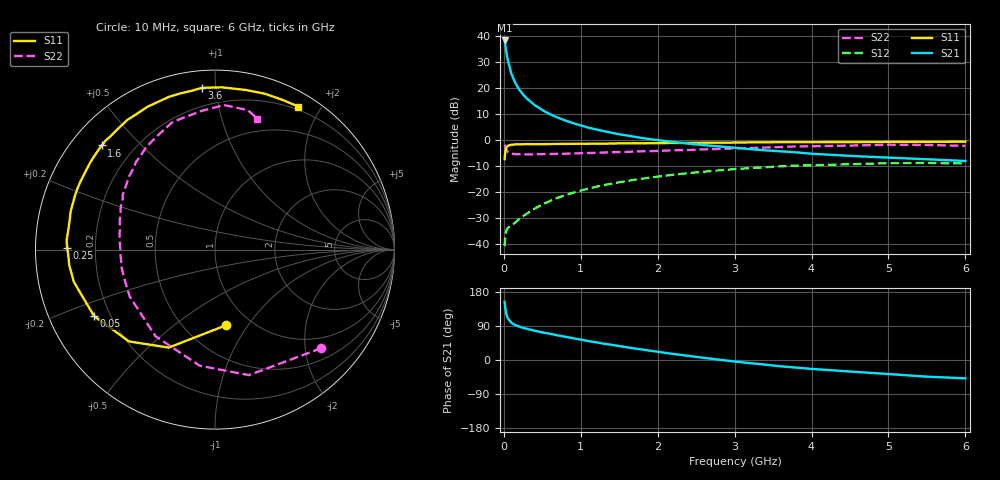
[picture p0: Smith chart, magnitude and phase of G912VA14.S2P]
! SIEMENS Small Signal Semiconductors
! BFG235
! Si NPN RF Bipolar Junction Transistor in SOT223
! VCE = 12 V  IC = 140 mA
! Common Emitter S-Parameters:  July  1994
# GHz  S  MA  R  50
!  f  S11  S21  S12  S22
! GHz  MAG  ANG  MAG  ANG  MAG  ANG  MAG  ANG
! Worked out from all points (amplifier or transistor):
!   40 points, 10 MHz to 6 GHz, reference 50 ohm
!   highest |S21| = 38.2 dB at 10 MHz (marker M1)
!   |S21| within 3 dB of that: start of sweep to 25.21 MHz
!   unconditionally stable (mu >= 1): 467.7 MHz to 1.48 GHz
!   at 200 MHz: K = 0.79, MSG = 24.8 dB, |S12| = -30.4 dB
!   at 1.5 GHz: K = 1.00, MSG = 9.2 dB, |S12| = -16.3 dB
!   at 6 GHz: K = 0.89, MSG = 0.5 dB, |S12| = -9.1 dB
!   S11 on the Smith chart (normalised r, x): 10 MHz: 0.77, -0.79; 50 MHz: 0.14, -0.25; 250 MHz: 0.10, +0.01; 1.6 GHz: 0.09, +0.39; 3.6 GHz: 0.09, +0.92; 6 GHz: 0.16, +1.73
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0.01  0.4268 -82.1  80.89 153.6  0.0091 62.6  0.808 -42.8
0.02  0.6039 -115.3  64.58 135.2  0.0145 48.9  0.7244 -74.9
0.03  0.7009 -133.1  51.26 123.3  0.0176 41.7  0.6526 -97.5
0.05  0.7688 -151.2  34.48 110.4  0.0202 33.9  0.5854 -124.5
0.1  0.8067 -167.1  18.29 98.0  0.023 36.4  0.5423 -151.3
0.15  0.8168 -174.0  12.31 91.9  0.026 42.5  0.5306 -162.5
0.2  0.8179 -177.8  9.214 88.1  0.0302 46.7  0.5299 -168.5
0.25  0.8239 179.2  7.422 84.9  0.0342 50.9  0.5269 -172.5
0.3  0.8285 176.5  6.195 82.3  0.0384 54.0  0.5272 -175.8
0.4  0.8246 171.9  4.659 77.3  0.0478 57.4  0.5273 179.8
0.5  0.8261 168.4  3.72 72.9  0.0573 59.0  0.5312 176.3
0.6  0.8318 165.2  3.105 69.2  0.0672 59.7  0.535 173.2
0.7  0.8333 161.6  2.674 64.9  0.0772 59.7  0.5394 170.4
0.9  0.8384 156.1  2.091 57.4  0.0966 57.9  0.5469 165.8
1.1  0.8417 149.7  1.714 49.8  0.116 55.7  0.559 161.2
1.6  0.8574 137.4  1.212 33.6  0.1624 47.6  0.5868 151.1
2.2  0.872 124.1  0.911 16.0  0.2134 36.9  0.6289 139.5
3.2  0.8914 102.8  0.665 -8.3  0.2863 17.6  0.6972 120.7
3.6  0.904 94.7  0.602 -16.7  0.3096 9.2  0.7287 112.3
4.5  0.9057 79.1  0.492 -30.4  0.3398 -7.2  0.776 95.6
5.5  0.9149 65.8  0.424 -44.0  0.3606 -25.6  0.7986 76.8
6  0.9222 59.8  0.393 -48.3  0.3506 -32.4  0.7669 72.1
